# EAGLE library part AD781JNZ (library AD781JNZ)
Sample and Hold Amplifier Check prices
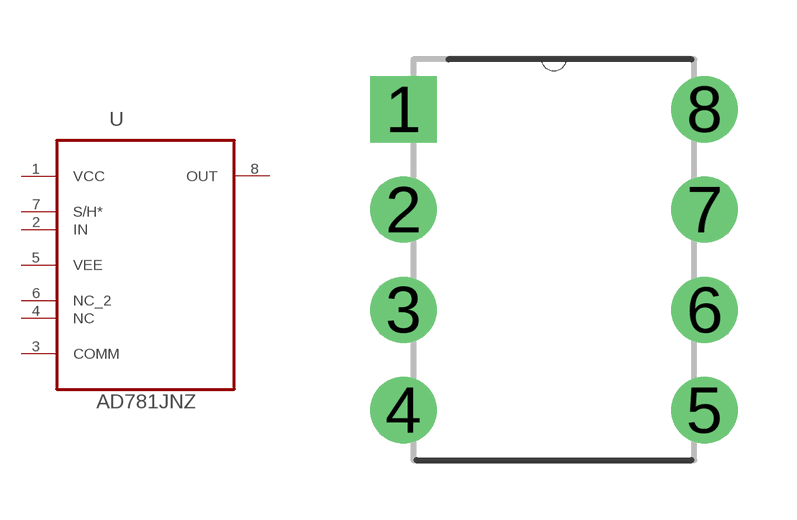
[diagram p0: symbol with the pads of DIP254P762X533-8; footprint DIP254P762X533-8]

Designator prefix U

## AD781JNZ (Availability: Good; Description: Sample and Hold Amplifier 1 Circuit 8-PDIP; MF: Analog Devices; MP: AD781JNZ; Package: PDIP-8 Analog Devices; Price: None; Purchase-URL: https://pricing.snapeda.com/search/part/AD781JNZ/?ref=eda)  [DIP254P762X533-8]
1  VCC  pwr
2  IN  in
3  COMM  pas
4  NC  nc
5  VEE  pwr
6  NC_2  nc
7  S/H*  pas
8  OUT  out

## Footprint DIP254P762X533-8 (pad centres in mm)
drill 1.118 square: 1 -7.62,7.62
drill 1.118: 2 -7.62,5.08; 3 -7.62,2.54; 4 -7.62,0; 5 0,0; 6 0,2.54; 7 0,5.08; 8 0,7.62

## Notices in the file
This work is licensed under a Creative Commons Attribution-ShareAlike 4.0 International License (CC BY-SA) with Design Exception 1.0
